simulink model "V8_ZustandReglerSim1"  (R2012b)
settings: Solver=ode45  SolverMode=SingleTasking  StartTime=0.0  StopTime=10  RelTol=1e-3
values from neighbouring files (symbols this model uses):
  A = [1 1    [V8_1_ZustandRegler.m]    (also in V8_2_ZustandRegler.m; V8_2_ZustandRegler_dist.m; V8_3_ZustandRegler.m = [-1, 0, 0; V8_5_ZustandRegler.m)
  B = [0; 1]    [V8_1_ZustandRegler.m]    (also in V8_2_ZustandRegler.m; V8_2_ZustandRegler_dist.m; V8_3_ZustandRegler.m = [1; 0; 0]; V8_5_ZustandRegler.m)
  F = place(A,B,pd)    [V8_1_ZustandRegler.m]    (also in V8_2_ZustandRegler.m; V8_2_ZustandRegler_dist.m; V8_3_ZustandRegler.m = S_c_n' * PA; V8_5_ZustandRegler.m)

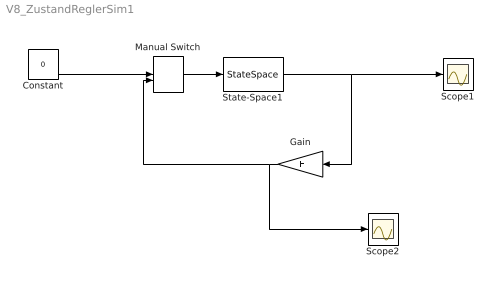
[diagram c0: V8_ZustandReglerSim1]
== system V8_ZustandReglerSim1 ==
  Constant : Constant  Value=0
  Gain : Gain  Gain=-F  Multiplication=Matrix(K*u)
  Manual Switch : ManualSwitch
  Scope1 : Scope
  Scope2 : Scope
  State-Space1 : StateSpace  A=A  B=B  C=eye(2)  D=[0; 0]  X0=[2; 2]  ContinuousStateAttributes='state_controller'
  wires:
  Gain/1 -> Manual Switch/2, Scope2/1
  Manual Switch/1 -> State-Space1/1
  State-Space1/1 -> Scope1/1, Gain/1
  Constant/1 -> Manual Switch/1
